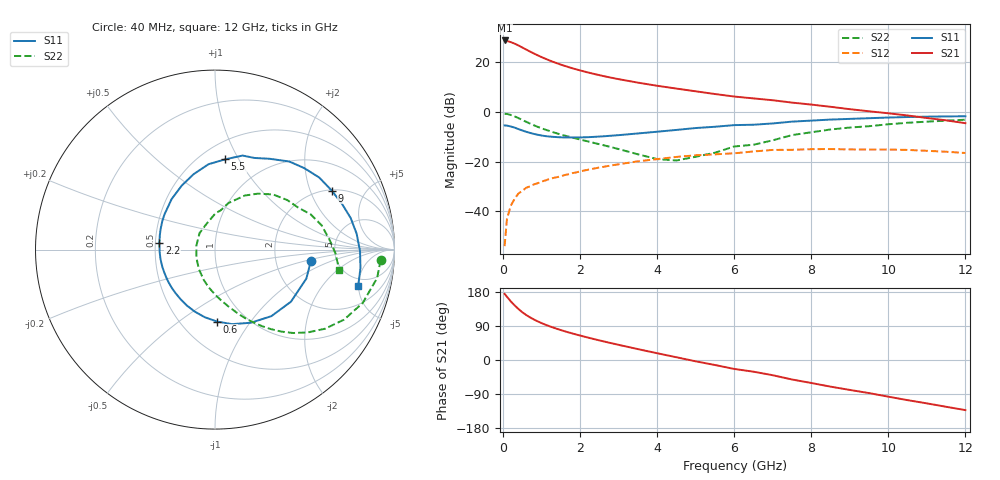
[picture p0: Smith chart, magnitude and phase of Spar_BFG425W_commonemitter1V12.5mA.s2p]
! Filename: 112bfg425.001
! BFG425W Field C1
! V1=8.600E-001V,V2=1.000E+000V, I1=1.841E-004A, I2=1.249E-002A
# GHz  S  MA  R 50
!  S11  S21  S12  S22
!Freq(GHz)  Mag  Ang  Mag  Ang  Mag  Ang  Mag  Ang
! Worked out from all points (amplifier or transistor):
!   44 points, 40 MHz to 12 GHz, reference 50 ohm
!   highest |S21| = 28.8 dB at 40 MHz (marker M1)
!   |S21| within 3 dB of that: start of sweep to 520.1 MHz
!   unconditionally stable (mu >= 1): 1.6 GHz to end of sweep
!   at 700 MHz: K = 0.63, MSG = 27.1 dB, |S12| = -29.9 dB
!   at 2.4 GHz: K = 1.14, MAG = 16.6 dB, |S12| = -22.6 dB
!   at 12 GHz: K = 1.37, MAG = 2.3 dB, |S12| = -16.5 dB
!   S11 on the Smith chart (normalised r, x): 40 MHz: 3.22, -0.57; 600 MHz: 0.74, -0.70; 2.2 GHz: 0.53, +0.04; 5.5 GHz: 0.65, +0.88; 9 GHz: 2.03, +2.86; 12 GHz: 3.95, -4.95
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0.04  0.538 -6.7  27.6 174.5  0.002 82.4  0.925 -3.6
0.1  0.534 -17.6  26.96 167.0  0.007 81.7  0.917 -10.0
0.2  0.513 -34.5  25.55 154.7  0.013 74.6  0.875 -19.9
0.3  0.486 -49.7  23.82 144.1  0.018 69.1  0.818 -28.5
0.4  0.454 -63.8  21.85 134.5  0.023 63.7  0.755 -35.7
0.5  0.426 -77.1  19.92 125.9  0.026 59.9  0.693 -41.8
0.6  0.401 -88.4  18.1 118.8  0.03 57.1  0.637 -46.8
0.7  0.381 -98.6  16.49 112.6  0.032 54.7  0.586 -51.2
0.9  0.349 -116.6  13.85 101.9  0.037 51.7  0.504 -58.1
1  0.337 -124.3  12.75 97.3  0.04 50.5  0.471 -61.1
1.2  0.322 -138.1  10.98 89.2  0.045 48.6  0.417 -66.3
1.6  0.309 -160.8  8.5 75.8  0.054 45.4  0.336 -75.2
2.2  0.312 172.9  6.273 59.3  0.069 40.0  0.257 -88.5
3  0.343 145.2  4.592 40.0  0.089 30.9  0.18 -110.4
3.5  0.371 130.7  3.91 28.7  0.102 24.3  0.141 -129.6
4.5  0.437 105.8  2.969 7.3  0.125 9.7  0.106 168.7
5.5  0.506 83.6  2.306 -13.2  0.141 -5.7  0.152 107.6
6.5  0.556 66.7  1.883 -30.9  0.161 -18.0  0.22 82.0
8.5  0.706 34.7  1.277 -70.3  0.18 -53.9  0.446 43.6
9  0.729 26.8  1.142 -79.0  0.177 -61.8  0.488 34.5
10.5  0.794 6.4  0.853 -106.0  0.173 -87.3  0.609 12.9
12  0.823 -14.2  0.597 -132.2  0.15 -115.4  0.702 -9.5
